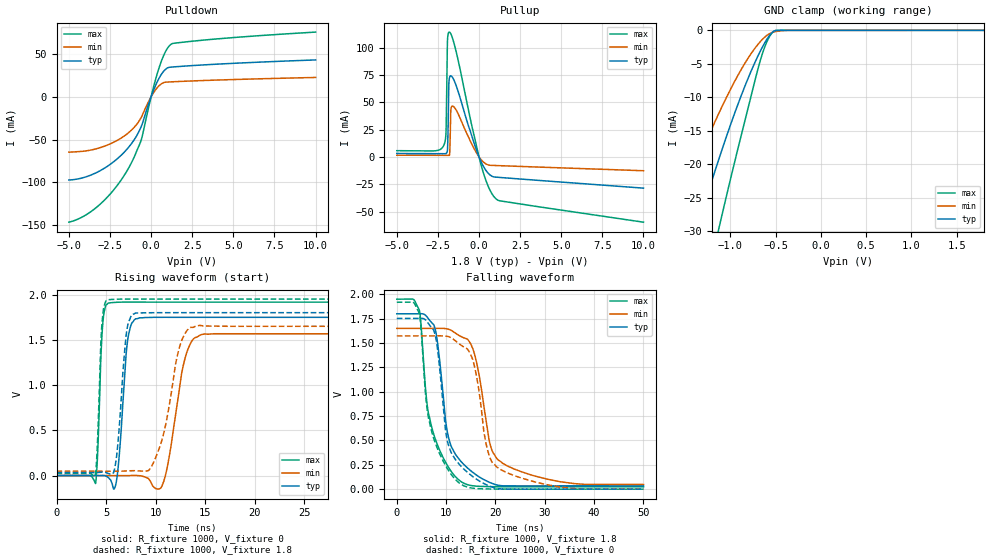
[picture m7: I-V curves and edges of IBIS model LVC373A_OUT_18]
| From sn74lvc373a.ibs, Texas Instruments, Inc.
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[Model]   LVC373A_OUT_18
Model_type  3-state
Enable   Active-Low
Vref =   0
Rref =   1000
Cref =   30p
Vmeas =   0.9
| variable   typ   min   max
C_comp   3.38pF   2.95pF   3.91pF
| C_pullup   10.53pF   0.66pF   30.94pF
| C_pulldown   6.52pF   3.18pF   9.18pF
| C_tri-state   3.38pF   2.95pF   3.91pF
[Temperature Range]   40   100   -40
| Ambient temperature   25   85   -40
[Voltage range]   1.8   1.65   1.95
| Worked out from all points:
|   slope of the pulldown table from 0 to 0.27 V, typ, clamps not added: 20.5 ohm
|   slope of the pullup table from 0 to 0.27 V, typ, clamps not added: 31.1 ohm
|   GND clamp passes 1 mA (typ) near -0.58 V on its own axis
|   rising waveform, R_fixture 1000, V_fixture 0: 20-80 % time 652ps typ, 1.34ns min, 377ps max; typ from 0 V to 1.75 V
|   falling waveform, R_fixture 1000, V_fixture 1.8: 20-80 % time 3.17ns typ, 3.55ns min, 3.52ns max; typ from 1.8 V to 0.033 V
|   rising waveform, R_fixture 1000, V_fixture 1.8: 20-80 % time 715ps typ, 1.63ns min, 370ps max; typ from 0.033 V to 1.8 V
|   falling waveform, R_fixture 1000, V_fixture 0: 20-80 % time 2.98ns typ, 3.19ns min, 3.43ns max; typ from 1.75 V to 0 V
[GND Clamp]
| LVC373A_OUT_18
|   Voltage   I(typ)   I(min)   I(max)
-5V       -227.5mA   -167.1mA   -315.1mA
-1.635V   -42.01mA   -28.83mA   -61.5mA
-1.37V    -29.68mA   -19.86mA   -44.35mA
-1.32V    -27.45mA   -18.25mA   -41.22mA
-1.135V   -19.53mA   -12.6mA    -30.03mA
-1.09V    -17.7mA    -11.31mA   -27.4mA
-860mV    -9.029mA   -5.369mA   -14.59mA
-670mV    -3.114mA   -1.689mA   -4.511mA
-590mV    -1.19mA    -686uA     -1.49mA
-520mV    -140.4uA   -252.6uA   -137.6uA
-330mV    -83.49nA   -2.853uA   -11.92nA
1.8V      12.9pA     11.43nA    4.783pA
[Pulldown]
| LVC373A_OUT_18
|   Voltage   I(typ)   I(min)   I(max)
-5V       -97.22mA   -64.67mA   -146.5mA
-4.07V    -94.17mA   -63.46mA   -139.2mA
-3.115V   -86.49mA   -59.52mA   -125.7mA
-2.2V     -74.72mA   -52.34mA   -107mA
-1.405V   -59.81mA   -42.45mA   -84.52mA
-950mV    -47.8mA    -33.93mA   -66.83mA
-600mV    -34.74mA   -24.02mA   -50.37mA
55mV      2.896mA    1.848mA    4.357mA
460mV     20.83mA    12.48mA    32.44mA
840mV     31.43mA    16.99mA    51.42mA
1.195V    34.65mA    17.43mA    61.13mA
10V       43.1mA     22.61mA    75.61mA
[Pullup]
| LVC373A_OUT_18
|   Voltage   I(typ)   I(min)   I(max)
-5V       3.151mA    1.569mA    5.717mA
-2.135V   2.927mA    1.444mA    10.77mA
-2.005V   3.14mA     1.435mA    23.85mA
-1.915V   6.909mA    1.428mA    107.3mA
-1.835V   66.2mA     1.419mA    114mA
-1.8V     72.1mA     1.42mA     114.2mA
-1.77V    73.52mA    8.583mA    113.9mA
-1.715V   74.22mA    42.42mA    112.6mA
-1.595V   72.39mA    46.51mA    107.8mA
105mV     -3.729mA   -2.103mA   -6.182mA
995mV     -18.46mA   -7.86mA    -37.84mA
10V       -28.56mA   -12.64mA   -59.72mA
[Ramp]
| LVC373A_OUT_18
| variable   typ   min   max
dV/dt_r   1.14/7.30E-10   1.03/1.53E-09   1.20/4.17E-10
dV/dt_f   1.06/3.24E-09   0.96/3.74E-09   1.16/3.56E-09
R_load = 1000
[Rising Waveform]
| LVC373A_OUT_18
R_fixture =   1000
C_fixture =   0
L_fixture =   0
V_fixture =   0
V_fixture_min = 0
V_fixture_max = 0
|   Time   V(typ)   V(min)   V(max)
0s        169pV      6.385nV    113.5pV
3.935ns   -821.5uV   48.2uV     -88.12mV
4.635ns   821uV      67.94uV    1.632V
5.24ns    -23.42mV   -376.2uV   1.906V
6.04ns    -66.1mV    -697.3uV   1.914V
7.135ns   1.458V     -1.01mV    1.917V
8ns       1.733V     1.099mV    1.917V
10.66ns   1.749V     -110.5mV   1.916V
14.64ns   1.748V     1.559V     1.916V
50ns      1.749V     1.566V     1.917V
[Falling Waveform]
| LVC373A_OUT_18
R_fixture =   1000
C_fixture =   0
L_fixture =   0
V_fixture =   1.8
V_fixture_min = 1.65
V_fixture_max = 1.95
|   Time   V(typ)   V(min)   V(max)
0s        1.8V       1.65V      1.95V
4.605ns   1.8V       1.65V      1.83V
6.1ns     1.77V      1.65V      890.4mV
7.48ns    1.689V     1.65V      565mV
10.28ns   578.3mV    1.644V     241.5mV
12.79ns   296.9mV    1.572V     85.89mV
15.57ns   166.2mV    1.418V     34.09mV
18.76ns   70.35mV    491.8mV    26.29mV
20.61ns   39.79mV    297.5mV    24.96mV
50ns      33.42mV    47.74mV    24.14mV
[Rising Waveform]
| LVC373A_OUT_18
R_fixture =   1000
C_fixture =   0
L_fixture =   0
V_fixture =   1.8
V_fixture_min = 1.65
V_fixture_max = 1.95
|   Time   V(typ)   V(min)   V(max)
0s        33.31mV    47.53mV    24.11mV
3.93ns    33.44mV    47.56mV    12.71mV
4.575ns   37.07mV    47.52mV    1.664V
5.21ns    22.59mV    47.28mV    1.942V
5.935ns   116.4mV    47.83mV    1.948V
7.045ns   1.566V     51.03mV    1.95V
7.955ns   1.795V     53.51mV    1.95V
10.29ns   1.8V       277.2mV    1.95V
13.53ns   1.8V       1.637V     1.95V
50ns      1.8V       1.65V      1.95V
[Falling Waveform]
| LVC373A_OUT_18
R_fixture =   1000
C_fixture =   0
L_fixture =   0
V_fixture =   0
V_fixture_min = 0
V_fixture_max = 0
|   Time   V(typ)   V(min)   V(max)
0s        1.752V     1.573V     1.918V
4.605ns   1.753V     1.573V     1.795V
6.04ns    1.726V     1.573V     867.7mV
7.465ns   1.634V     1.573V     524mV
10.17ns   515.4mV    1.569V     218.7mV
12.71ns   252mV      1.489V     61.59mV
15.41ns   128.9mV    1.328V     10.25mV
18.23ns   43.71mV    436.8mV    2.545mV
20.4ns    6.419mV    222.1mV    881.4uV
50ns      108.5uV    187.8uV    25.54uV
